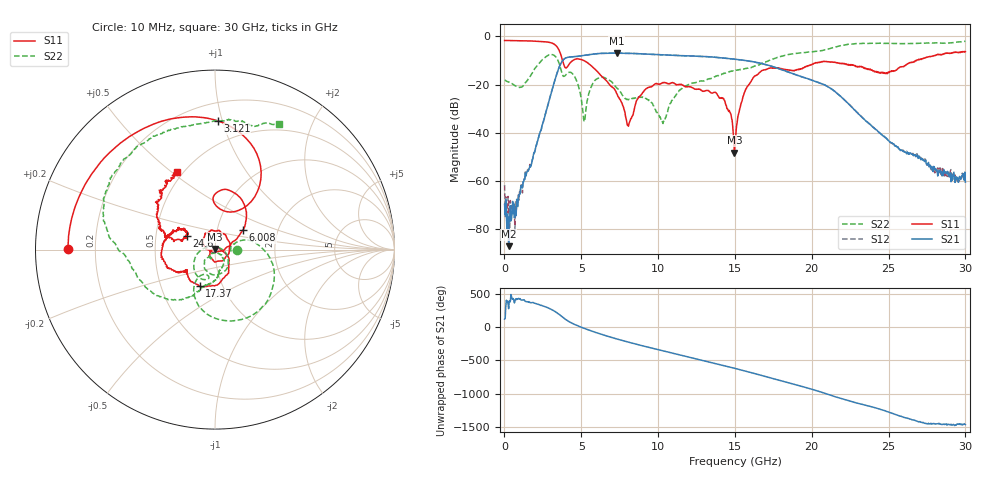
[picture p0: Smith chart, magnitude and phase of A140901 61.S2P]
!  2-Port S-parameters saved by WinCal
! VAR MeasName=S-Parameters (CALIBRATED_DATA) read from VNA (N5244A)
! VAR MeasDate=11/3/2014 9:36:44 AM
! VAR NAME=A140901 61
! VAR FILENAME=A140901 61.S2P
! VAR DATE=11/3/2014 9:36:44 AM
! VAR PHYS_PORTS=1,2
# Hz S RI R 50
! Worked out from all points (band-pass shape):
!   801 points, 10 MHz to 30 GHz, reference 50 ohm
!   highest |S21| = -6.98 dB at 7.32 GHz (marker M1); lowest = -86.9 dB at 272.4 MHz (marker M2)
!   |S21| within 3 dB of the highest: 3.796 GHz to 15.62 GHz (11.82 GHz wide, 122 % of centre)
!   lowest |S11| = -48.2 dB at 14.97 GHz (marker M3), VSWR 1.01, Z = 49.9 + j0.372 ohm
!   |S11| at or under -10 dB: 3.781 GHz to 4.456 GHz (675.4 MHz wide, 16.4 % of centre); 5.154 GHz to 26.83 GHz (21.67 GHz wide, 136 % of centre)
!   |S22| runs from -36.1 to -2.1 dB; largest |S21 - S12| = 0.0019
!   S11 on the Smith chart (normalised r, x): 10 MHz: 0.10, +0.00; 3.121 GHz: 0.33, +0.97; 6.008 GHz: 1.33, +0.31; 17.37 GHz: 0.78, -0.33; 24.6 GHz: 0.72, +0.12; 30 GHz: 0.47, +0.52
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1e7  -0.8195 0.00326  -0.000188 0.000272  2.73e-05 0.000828  0.1242 -0.000924
2.724125e8  -0.8141 0.0886  9.7e-06 -4.39e-05  2e-05 0.00035  0.1113 -0.0133
7.972375e8  -0.7727 0.2558  0.000221 0.000358  8.95e-05 0.000278  0.0905 -0.0101
3.121462e9  0.0153 0.7174  -0.0108 -0.0819  -0.0108 -0.0817  0.1476 -0.3892
3.75875e9  0.2014 0.2674  -0.2855 0.1087  -0.2849 0.1081  -0.0812 -0.145
4.2086e9  -0.00681 0.2638  0.0243 0.3699  0.0241 0.3697  -0.0689 -0.166
5.033325e9  0.1286 0.3006  0.3954 -0.00685  0.3953 -0.00639  -0.0397 0.0148
5.25825e9  0.1595 0.2576  0.3796 -0.1442  0.3796 -0.1437  0.0198 0.0116
6.008e9  0.157 0.1107  0.0594 -0.4312  0.0599 -0.4311  0.0567 -0.1172
7.320062e9  0.0634 0.0107  -0.4463 -0.034  -0.4453 -0.035  -0.0584 -0.0612
8.1073e9  -0.00319 -0.0153  -0.3091 0.3163  -0.3095 0.3162  -0.023 -0.0439
1.001916e10  -0.0456 0.092  0.3871 0.1551  0.3862 0.1551  -0.0139 -0.0198
1.208098e10  0.0828 0.035  -0.0173 -0.3913  -0.0167 -0.3911  0.0422 -0.0936
1.421776e10  -0.0351 -0.0388  -0.2938 0.2004  -0.2944 0.2004  0.00384 -0.166
1.496751e10  -0.00118 0.00373  -0.0693 0.3283  -0.0683 0.3281  -0.0334 -0.1915
1.5005e10  0.00166 0.00588  -0.0568 0.3298  -0.0559 0.3288  -0.033 -0.193
1.575475e10  0.0737 -0.0416  0.1805 0.2552  0.1794 0.2546  -0.0649 -0.2056
1.736671e10  -0.0857 -0.2033  0.1638 -0.176  0.1641 -0.1751  -0.1761 -0.2772
2.002832e10  -0.2382 -0.1116  -0.0979 0.0737  -0.0986 0.0733  -0.4671 -0.0873
2.46018e10  -0.155 0.0774  -0.00877 -0.00185  -0.00886 -0.00182  -0.3286 0.6355
2.501416e10  -0.1632 0.0646  -0.00637 0.00255  -0.00642 0.00245  -0.2613 0.6649
3e10  -0.2091 0.4325  0.000827 -0.000472  0.001 -0.000846  0.3587 0.6976
